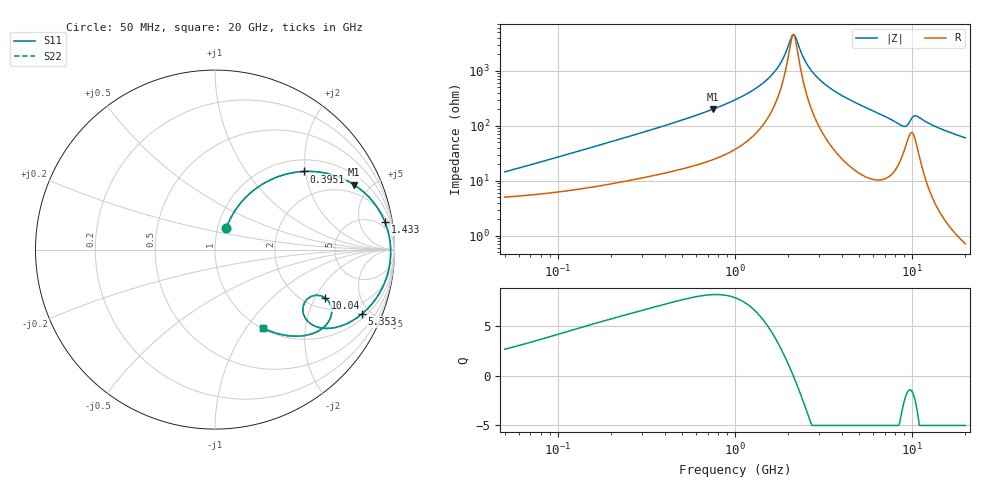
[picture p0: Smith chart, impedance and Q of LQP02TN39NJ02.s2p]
!Murata Part Number: LQP02TN39NJ02
!These Parameters are Measured in Series Mode Connection
!  o--[Z]--o
!Port1  Port2
!  o-------o
!Freq. Start=50[MHz] Stop=20[GHz], 401[Steps]
# Hz S RI R 50
!Freq.(Hz) S11(Real) S11(Imag) S21(Real) S21(Imag) S12(Real) S12(Imag) S22(Real) S22(Imag)
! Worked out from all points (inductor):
!   401 points, 50 MHz to 20 GHz, reference 50 ohm
!   read as one part in series: L = 42.4 nH near 58.96 MHz
!   highest Q = 8.22 at 752.3 MHz (marker M1), where L = 42.1 nH
!   self-resonance near 2.115 GHz
!   S11 on the Smith chart (normalised r, x): 50 MHz: 1.10, +0.27; 395.1 MHz: 1.27, +1.96; 1.433 GHz: 3, +12; 5.353 GHz: 1.24, -4.43; 10.04 GHz: 2.49, -2.43; 20 GHz: 1.01, -1.20
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5e7  0.0636 0.1211  0.9364 -0.1211  0.9364 -0.1211  0.0636 0.1211
1.364002e8  0.1578 0.2769  0.8422 -0.2769  0.8422 -0.2769  0.1578 0.2769
3.721004e8  0.4701 0.4335  0.5299 -0.4335  0.5299 -0.4335  0.4701 0.4335
3.95076e8  0.4963 0.4354  0.5037 -0.4354  0.5037 -0.4354  0.4963 0.4354
7.523192e8  0.7744 0.3615  0.2256 -0.3615  0.2256 -0.3615  0.7744 0.3615
1e9  0.8691 0.28  0.1309 -0.28  0.1309 -0.28  0.8691 0.28
1.432596e9  0.9468 0.1535  0.0532 -0.1535  0.0532 -0.1535  0.9468 0.1535
1.766834e9  0.9704 0.0739  0.0296 -0.0739  0.0296 -0.0739  0.9704 0.0739
1.904239e9  0.9751 0.0449  0.0249 -0.0449  0.0249 -0.0449  0.9751 0.0449
2.083303e9  0.9783 0.00983  0.0217 -0.00983  0.0217 -0.00983  0.9783 0.00983
2.146657e9  0.9787 -0.00192  0.0213 0.00192  0.0213 0.00192  0.9787 -0.00192
2.211938e9  0.9788 -0.0137  0.0212 0.0137  0.0212 0.0137  0.9788 -0.0137
2.456456e9  0.9768 -0.0552  0.0232 0.0552  0.0232 0.0552  0.9768 -0.0552
2.728004e9  0.9709 -0.0969  0.0291 0.0969  0.0291 0.0969  0.9709 -0.0969
3.572216e9  0.9361 -0.2049  0.0639 0.2049  0.0639 0.2049  0.9361 -0.2049
5.352748e9  0.8183 -0.3591  0.1817 0.3591  0.1817 0.3591  0.8183 -0.3591
7.442007e9  0.6343 -0.439  0.3657 0.439  0.3657 0.439  0.6343 -0.439
9.041845e9  0.4893 -0.3391  0.5107 0.3391  0.5107 0.3391  0.4893 -0.3391
1.004137e10  0.614 -0.2689  0.386 0.2689  0.386 0.2689  0.614 -0.2689
1.082228e10  0.646 -0.3724  0.354 0.3724  0.354 0.3724  0.646 -0.3724
1.257102e10  0.539 -0.4696  0.461 0.4696  0.461 0.4696  0.539 -0.4696
2e10  0.2684 -0.4372  0.7316 0.4372  0.7316 0.4372  0.2684 -0.4372
